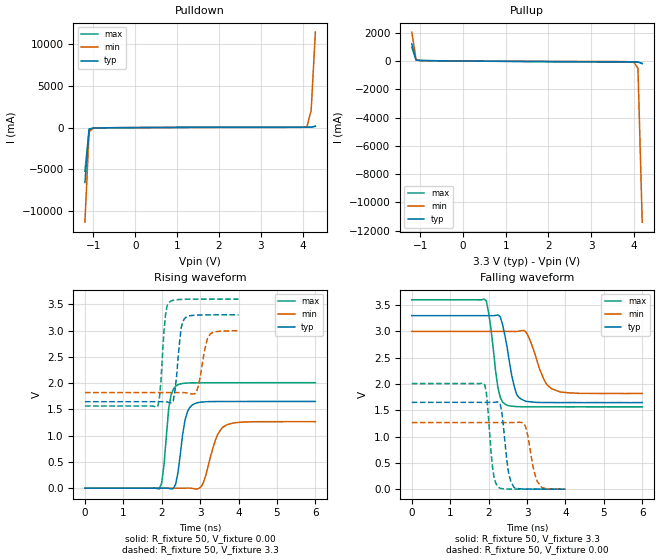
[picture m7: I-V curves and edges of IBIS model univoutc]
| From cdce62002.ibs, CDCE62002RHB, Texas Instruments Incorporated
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|   Model   univoutc
[Model]   univoutc
Model_type   Output
Polarity   Non-Inverting
Vmeas  =   1.55V
Cref   =   5pF
Vref   =   0V
|Variable   typ   min   max
C_comp   1.482e-12   1.466e-12   1.603e-12
[Model Spec]
Vmeas   1.55V   1.4V   1.7V
|Variable   typ   min   max
[Voltage range]   3.3   3.0   3.6
|Variable   typ   min   max
[Temperature range]  25   85   0
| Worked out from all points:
|   slope of the pulldown table from 0 to 0.495 V, typ, clamps not added: 41.5 ohm
|   slope of the pullup table from 0 to 0.495 V, typ, clamps not added: 45.4 ohm
|   rising waveform, R_fixture 50, V_fixture 0.00: 20-80 % time 187ps typ, 301ps min, 151ps max; typ from 0 V to 1.65 V
|   falling waveform, R_fixture 50, V_fixture 3.3: 20-80 % time 250ps typ, 349ps min, 202ps max; typ from 3.3 V to 1.65 V
|   rising waveform, R_fixture 50, V_fixture 3.3: 20-80 % time 130ps typ, 178ps min, 113ps max; typ from 1.65 V to 3.3 V
|   falling waveform, R_fixture 50, V_fixture 0.00: 20-80 % time 150ps typ, 198ps min, 134ps max; typ from 1.65 V to 0.001 V
[Pulldown]
|Voltage   I(typ)   I(min)   I(max)
-1.2V     -6.6A      -11.38A    -5.251A
-1.1V     -201.8mA   -492.4mA   -162.6mA
-1V       -58.65mA   -57.19mA   -74.14mA
3.9V      42.87mA    32.53mA    55.73mA
4.1V      48.1mA     118.5mA    56.63mA
4.2V      51.39mA    2.059A     59.27mA
4.3V      155.5mA    11.49A     162.7mA
[Pullup]
|Voltage   I(typ)   I(min)   I(max)
-1.2V     1.203A     2.045A     971.5mA
-1.1V     61.22mA    106.4mA    62.19mA
-1V       32.93mA    26.89mA    42.72mA
4V        -60.97mA   -75.5mA    -73.88mA
4.1V      -68.4mA    -511.2mA   -75.39mA
4.2V      -177.8mA   -11.4A     -179.9mA
[Ramp]
|Variable   typ   min   max
dV/dt_r  0.9909/1.816e-10   0.7602/3.000e-10   1.2053/1.405e-10
dV/dt_f  0.9926/2.376e-10   0.7090/3.449e-10   1.2215/1.947e-10
R_load  =  50
[Rising Waveform]
R_fixture   =   50
V_fixture   =   0.00
V_fixture_min   =   0.00
V_fixture_max   =   0.00
C_fixture   =   0.00
|Time   V(typ)   V(min)   V(max)
0s        0V         0V         0V
1.939ns   -43.98uV   0V         -12.84mV
2.061ns   897.5uV    0V         453.3mV
2.242ns   -14.76mV   2.158uV    1.771V
2.424ns   302.6mV    -45.91uV   1.971V
2.606ns   1.296V     879.2uV    1.998V
2.848ns   1.606V     -10.7mV    2.005V
3.03ns    1.639V     29.96mV    2.007V
3.697ns   1.65V      1.207V     2.008V
6ns       1.651V     1.266V     2.008V
[Falling Waveform]
R_fixture   =   50
V_fixture   =   3.3
V_fixture_min   =   3.0
V_fixture_max   =   3.6
C_fixture   =   0.00
|Time   V(typ)   V(min)   V(max)
0s        3.3V       3V         3.6V
1.939ns   3.3V       3V         3.584V
2.242ns   3.313V     3V         1.93V
2.364ns   3.128V     3V         1.655V
2.485ns   2.685V     3V         1.594V
2.727ns   1.804V     2.999V     1.571V
2.97ns    1.67V      2.992V     1.567V
3.455ns   1.649V     2.066V     1.565V
3.636ns   1.648V     1.912V     1.565V
6ns       1.647V     1.819V     1.565V
[Rising Waveform]
R_fixture   =   50
V_fixture   =   3.3
V_fixture_min   =   3.0
V_fixture_max   =   3.6
C_fixture   =   0.00
|Time   V(typ)   V(min)   V(max)
0s        1.646V     1.819V     1.565V
1.899ns   1.646V     1.819V     1.563V
2.101ns   1.644V     1.819V     3.316V
2.182ns   1.633V     1.819V     3.528V
2.303ns   1.669V     1.819V     3.578V
2.505ns   3.048V     1.82V      3.593V
2.586ns   3.223V     1.819V     3.595V
2.909ns   3.294V     1.843V     3.598V
3.273ns   3.299V     2.943V     3.599V
4ns       3.299V     2.998V     3.599V
[Falling Waveform]
R_fixture   =   50
V_fixture   =   0.00
V_fixture_min   =   0.00
V_fixture_max   =   0.00
C_fixture   =   0.00
|Time   V(typ)   V(min)   V(max)
0s        1.651V     1.267V     2.008V
1.859ns   1.651V     1.267V     2.021V
1.939ns   1.651V     1.267V     1.844V
2.101ns   1.651V     1.267V     420.3mV
2.222ns   1.659V     1.267V     65.11mV
2.303ns   1.616V     1.267V     15.81mV
2.667ns   31.19mV    1.267V     1.937mV
2.949ns   3.223mV    1.21V      1.208mV
3.273ns   1.281mV    138.8mV    720.6uV
4ns       592uV      1.436mV    329.7uV
